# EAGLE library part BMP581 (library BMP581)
Pressure Sensor 4.35PSI ~ 18.13PSI (30kPa ~ 125kPa) Absolute 10-WFLGA Source: Datasheet
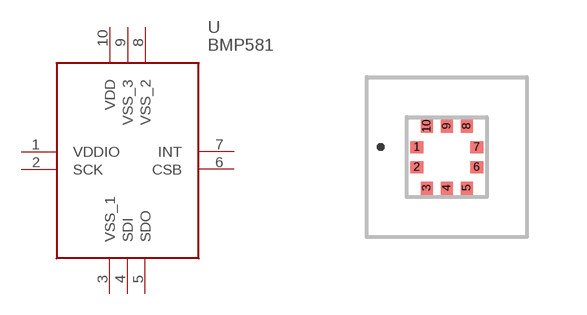
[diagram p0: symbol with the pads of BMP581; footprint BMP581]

Designator prefix U

## BMP581 (Arrow_Part_Number: BMP581; Arrow_Price-Stock: https://www.arrow.com/en/products/bmp581/bosch-sensortec?utm_currency=USD&region=nac; Description: Pressure Sensor 4.35PSI ~ 18.13PSI (30kPa ~ 125kPa) Absolute 10-WFLGA; Height: 0.8mm; Manufacturer_Name: BOSCH; Manufacturer_Part_Number: BMP581; Mouser_Part_Number: 262-BMP581; Mouser_Price-Stock: https://www.mouser.co.uk/ProductDetail/Bosch-Sensortec/BMP581?qs=Li%252BoUPsLEntPL9tlFmcgXg%3D%3D)  [BMP581]
1  VDDIO
2  SCK
3  VSS_1
4  SDI
5  SDO
6  CSB
7  INT
8  VSS_2
9  VSS_3
10  VDD

## Footprint BMP581 (pad centres in mm)
BMP581-7
smd 0.325 x 0.3: 1 -0.75,0.25; 2 -0.75,-0.25; 6 0.75,-0.25; 7 0.75,0.25
smd 0.3 x 0.325: 3 -0.5,-0.775; 4 0,-0.775; 5 0.5,-0.775; 8 0.5,0.775; 9 0,0.775; 10 -0.5,0.775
